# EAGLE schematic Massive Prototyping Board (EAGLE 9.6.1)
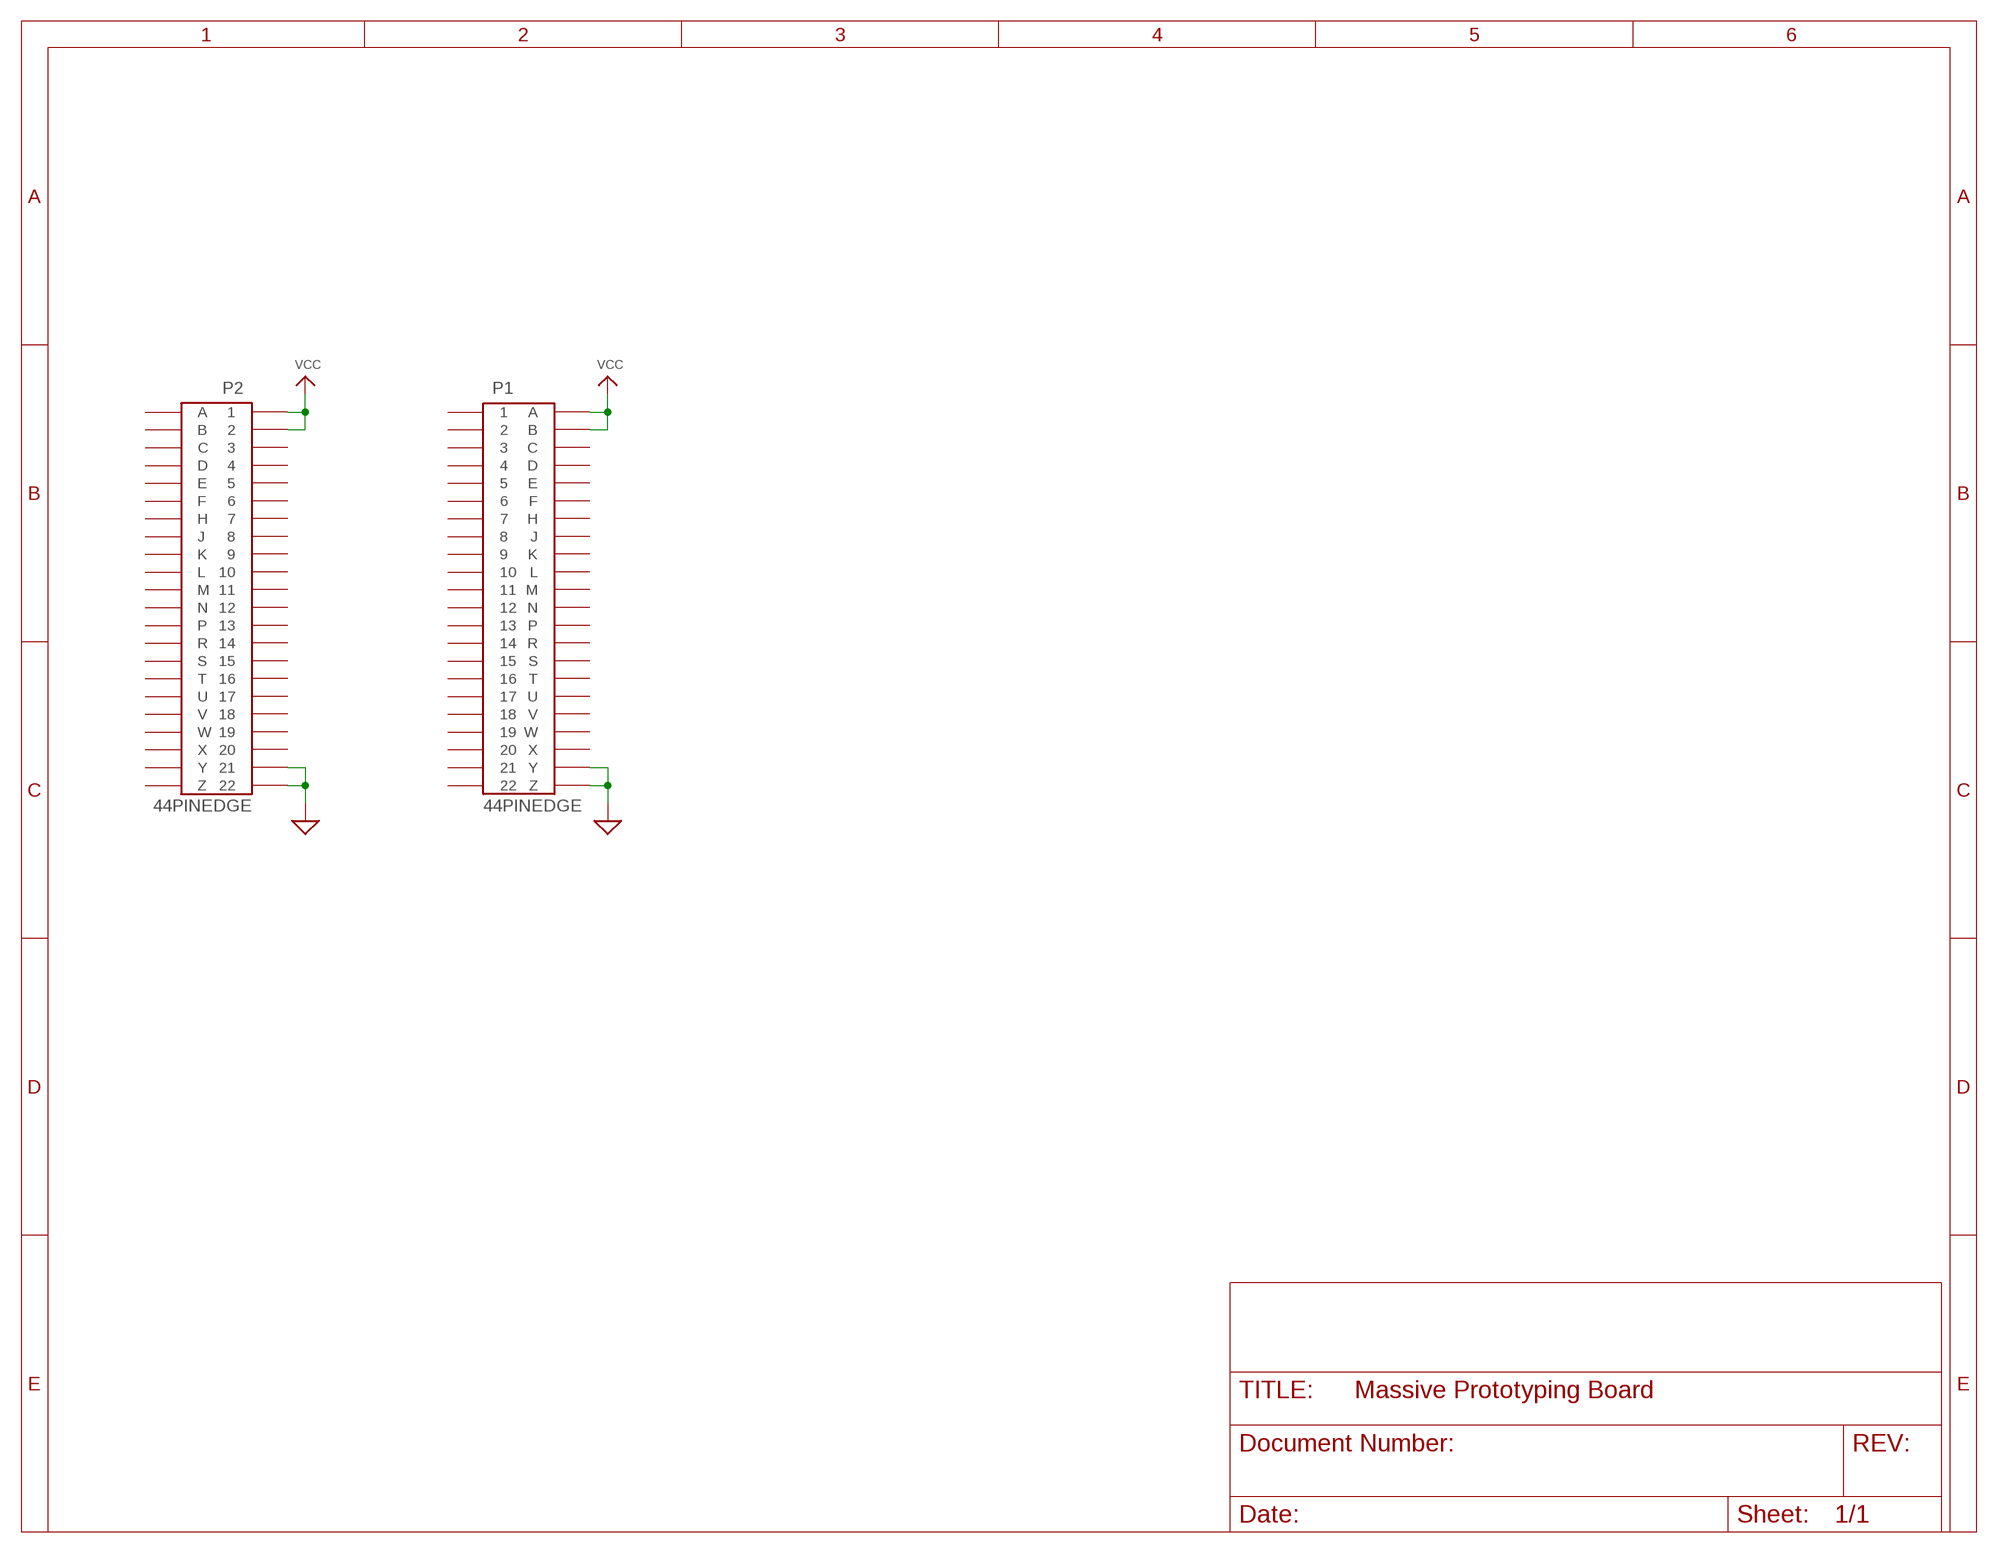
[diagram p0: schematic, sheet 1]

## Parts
P1  44PINEDGE  [44PINEDGE]
P2  44PINEDGE  [44PINEDGE]

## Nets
GND: P1.Y P1.Z P2.21 P2.22 ; supply symbol labelled SUP
VCC: P1.A P1.B P2.1 P2.2
Unconnected: P1.1 P1.2 P1.3 P1.4 P1.5 P1.6 P1.7 P1.8 P1.9 P1.10 P1.11 P1.12 P1.13 P1.14 P1.15 P1.16 P1.17 P1.18 P1.19 P1.20 P1.21 P1.22 P1.C P1.D P1.E P1.F P1.H P1.J P1.K P1.L P1.M P1.N P1.P P1.R P1.S P1.T P1.U P1.V P1.W P1.X P2.3 P2.4 P2.5 P2.6 P2.7 P2.8 P2.9 P2.10 P2.11 P2.12 P2.13 P2.14 P2.15 P2.16 P2.17 P2.18 P2.19 P2.20 P2.A P2.B P2.C P2.D P2.E P2.F P2.H P2.J P2.K P2.L P2.M P2.N P2.P P2.R P2.S P2.T P2.U P2.V P2.W P2.X P2.Y P2.Z

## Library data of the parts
P1 P2 = edge-156:44PINEDGE: 44 PIN EDGE CONNECTOR FOR PCB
